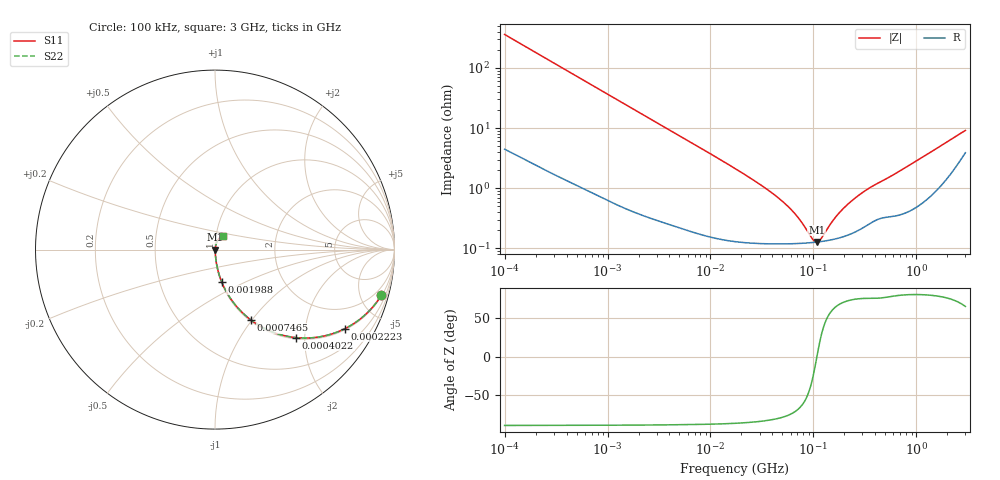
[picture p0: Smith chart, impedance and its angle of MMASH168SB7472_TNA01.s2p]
! MMASH168SB7472_TNA01  S-PARAMETER MODEL  ( Standard Model )
! Model Generated by TAIYO YUDEN Corporation (http://www.ty-top.com)
! Version 1.0
! TAIYO YUDEN Control No. 220601
! Copyright(c) 2013 TAIYO YUDEN CO.,LTD. All Rights Reserved.
! Product Description (link to TY-COMPAS)
! https://ds.yuden.co.jp/TYCOMPAS/or/detail?pn=MMASH168SB7472KTNA01&u=M
! Products Name : Multilayer Ceramic Capacitors
! Characteristics :
!  Capacitance : 4700 [pF] , Rated Voltage : 100 [V] , TCC : X7R
!  Case Size : 1.6 x 0.8 / 0.063 x 0.031 [mm/inch] , Thickness : 0.8 / 0.031 [mm/inch]
!  (Conditions: Temperature = 25 [degC] , DC Bias Voltage = 0 [V])
! External Node Assignments :
!  1  o---| |---o  2
! GND o---------o GND
! Frequency Range : 100kHz  -  3GHz  [ 401 STEP ]
# MHZ S RI R 50
! Freq[MHz].  S11 Real  S11 Imag  S21 Real  S21 Imag  S12 Real  S12 Imag  S22 Real  S22 Imag
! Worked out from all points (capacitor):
!   401 points, 100 kHz to 3 GHz, reference 50 ohm
!   read as one part in series: C = 4.4 nF near 105.3 kHz
!   lowest |Z| = 127 mohm at 108 MHz (marker M1)
!   series resonance near 108.3 MHz, so ESL is about 490 pH
!   S11 on the Smith chart (normalised r, x): 100 kHz: 1.09, -7.22; 222.3 kHz: 1.04, -3.27; 402.2 kHz: 1.03, -1.82; 746.5 kHz: 1.02, -0.98; 1.988 MHz: 1.01, -0.37; 3 GHz: 1.08, +0.17
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0.1  0.926 -0.2557  0.074 0.2557  0.074 0.2557  0.926 -0.2557
0.151038  0.8486 -0.352  0.1514 0.352  0.1514 0.352  0.8486 -0.352
0.222319  0.7248 -0.4399  0.2752 0.4399  0.2752 0.4399  0.7248 -0.4399
0.402172  0.4525 -0.4904  0.5475 0.4904  0.5475 0.4904  0.4525 -0.4904
0.562235  0.3007 -0.4509  0.6993 0.4509  0.6993 0.4509  0.3007 -0.4509
0.746515  0.1987 -0.391  0.8013 0.391  0.8013 0.391  0.1987 -0.391
1.156955  0.0963 -0.2863  0.9037 0.2863  0.9037 0.2863  0.0963 -0.2863
1.987766  0.0369 -0.1787  0.9631 0.1787  0.9631 0.1787  0.0369 -0.1787
3.161081  0.0164 -0.1154  0.9836 0.1154  0.9836 0.1154  0.0164 -0.1154
6.674626  0.00497 -0.0556  0.995 0.0556  0.995 0.0556  0.00497 -0.0556
17.7727  0.00171 -0.0206  0.9983 0.0206  0.9983 0.0206  0.00171 -0.0206
33.85116  0.00129 -0.0101  0.9987 0.0101  0.9987 0.0101  0.00129 -0.0101
52.46276  0.00122 -0.0055  0.9988 0.0055  0.9988 0.0055  0.00122 -0.0055
71.47675  0.00121 -0.00298  0.9988 0.00298  0.9988 0.00298  0.00121 -0.00298
97.38194  0.00125 -0.00074  0.9988 0.00074  0.9988 0.00074  0.00125 -0.00074
107.9567  0.00127 -2.18e-05  0.9987 2.18e-05  0.9987 2.18e-05  0.00127 -2.18e-05
119.6798  0.0013 0.000695  0.9987 -0.000695  0.9987 -0.000695  0.0013 0.000695
171.6802  0.00147 0.0033  0.9985 -0.0033  0.9985 -0.0033  0.00147 0.0033
222.1509  0.00171 0.00538  0.9983 -0.00538  0.9983 -0.00538  0.00171 0.00538
335.5313  0.00252 0.00928  0.9975 -0.00928  0.9975 -0.00928  0.00252 0.00928
547.5153  0.00355 0.0149  0.9965 -0.0149  0.9965 -0.0149  0.00355 0.0149
3000  0.0435 0.0761  0.9565 -0.0761  0.9565 -0.0761  0.0435 0.0761
